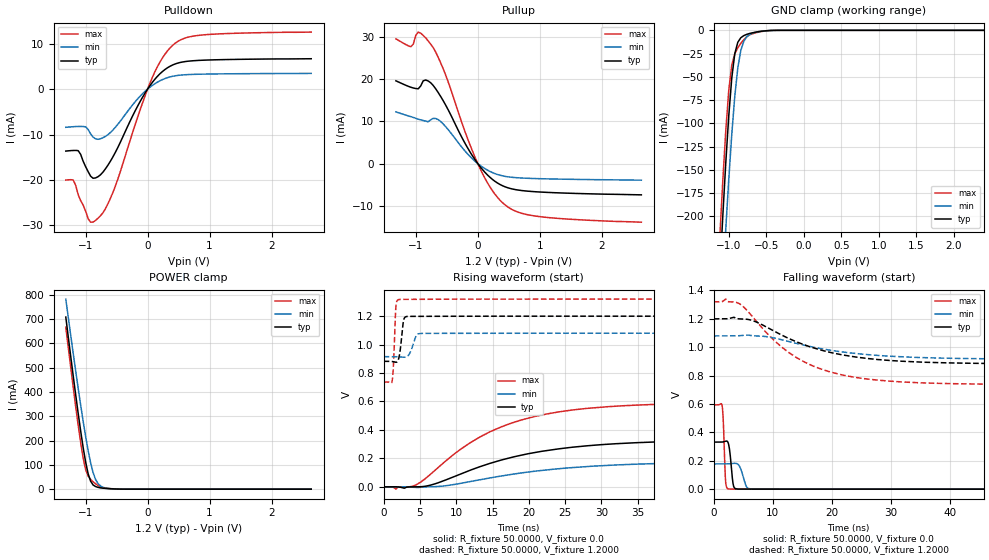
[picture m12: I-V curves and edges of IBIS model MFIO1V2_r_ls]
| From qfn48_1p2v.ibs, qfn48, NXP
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[Model] MFIO1V2_r_ls
|   Model MFIO1V2_r_ls
| This model was characterised for following simulation conditions:
| External (pad) voltage:
|   - Typ: 1.2V,   - Min: 1.08V,   - Max: 1.32V
| Library cells for typ/min/max conditions are connected as defined below:
|  IO - External Pad
|  A - Core Input
|  EN - Output Buffer Enable
|  BOOST - vdde
|  EHS - gnd
|  ENZI - vdd
|  EPD - vdd
|  EPUN - gnd
|  ZI - NC
|  ZIF - NC
|  gnd - gnd
|  gnde - gnde
|  vdd - vdd
|  vdde - vdde
| All other pins connected to ground
Model_type I/O
Polarity   Non-Inverting
Enable   Active-Low
Vinl =   0.3600V
Vinh =   0.8400V
Vmeas =  0.6000V
Cref =   20.0000F
Rref =   1.0000M
Vref =   0.0V
C_comp   1.6368pF   1.5495pF   1.7159pF
|C_comp_pullup   0.8309pF   0.8676pF   0.7830pF
|C_comp_pulldown   0.5929pF   0.6311pF   0.5574pF
[Model Spec]
| variable   typ   min   max
Vinh   0.3600V   0.3240V   0.3960V
Vinl   0.8400V   0.7560V   0.9240V
Vmeas   0.6000V   0.5400V   0.6600V
[Temperature Range]   25.0000   0.1250k   -40.0000
[Voltage Range]   1.2000V   1.0800V   1.3200V
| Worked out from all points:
|   slope of the pulldown table from 0 to 0.18 V, typ, clamps not added: 58.2 ohm
|   slope of the pullup table from 0 to 0.18 V, typ, clamps not added: 59.4 ohm
|   GND clamp passes 1 mA (typ) near -0.56 V on its own axis
|   POWER clamp passes 1 mA (typ) near -0.54 V on its own axis
|   rising waveform, R_fixture 50.0000, V_fixture 0.0: 20-80 % time 14.4ns typ, 16.1ns min, 12.2ns max; typ from 0 V to 0.331 V
|   rising waveform, R_fixture 50.0000, V_fixture 1.2000: 20-80 % time 407ps typ, 670ps min, 259ps max; typ from 0.882 V to 1.2 V
|   falling waveform, R_fixture 50.0000, V_fixture 0.0: 20-80 % time 465ps typ, 791ps min, 298ps max; typ from 0.331 V to 0 V
|   falling waveform, R_fixture 50.0000, V_fixture 1.2000: 20-80 % time 12.6ns typ, 13.9ns min, 10.9ns max; typ from 1.2 V to 0.882 V
[Pulldown]
|Voltage   I(typ)   I(min)   I(max)
-1.32V    -13.65mA   -8.413mA   -20.02mA
-1.2V     -13.51mA   -8.286mA   -20.01mA
-1.12V    -13.55mA   -8.228mA   -23.23mA
-920mV    -19.16mA   -9.849mA   -29.29mA
-720mV    -18.27mA   -10.7mA    -27.21mA
-520mV    -13.92mA   -8.406mA   -21.33mA
-160mV    -3.727mA   -2.148mA   -6.154mA
80mV      1.535mA    840.4uA    2.681mA
280mV     4.299mA    2.312mA    7.674mA
480mV     5.684mA    2.989mA    10.42mA
960mV     6.383mA    3.3mA      11.99mA
2.64V     6.67mA     3.446mA    12.53mA
[Pullup]
|Voltage   I(typ)   I(min)   I(max)
-1.32V    19.64mA    12.26mA    29.6mA
-1.08V    18.12mA    11.13mA    27.73mA
-960mV    17.74mA    10.54mA    31.21mA
-840mV    19.83mA    10.07mA    29.84mA
-720mV    18.57mA    10.71mA    27.56mA
-520mV    13.94mA    8.794mA    21.09mA
-200mV    4.663mA    2.883mA    7.362mA
40mV      -771.3uA   -452.7uA   -1.28mA
240mV     -3.804mA   -2.171mA   -6.507mA
480mV     -5.732mA   -3.143mA   -10.26mA
1.04V     -6.794mA   -3.614mA   -12.68mA
2.64V     -7.439mA   -3.951mA   -13.93mA
[GND_clamp]
|Voltage   I(typ)   I(min)   I(max)
-1.32V    -596.2mA   -647.7mA   -564.2mA
-1.12V    -261.7mA   -329.6mA   -222.8mA
-1.08V    -200.1mA   -270.2mA   -162.2mA
-1.04V    -142.4mA   -213.4mA   -108mA
-1V       -91.66mA   -160.1mA   -64.4mA
-960mV    -51.26mA   -111.8mA   -37.36mA
-920mV    -25.17mA   -71.04mA   -25.19mA
-880mV    -12.89mA   -40.68mA   -18.85mA
-800mV    -5.7mA     -11.79mA   -10.05mA
-680mV    -2.586mA   -2.926mA   -3.538mA
-440mV    -160.8uA   -186.1uA   -197.3uA
2.64V     0A         0A         0A
[POWER_clamp]
|Voltage   I(typ)   I(min)   I(max)
-1.32V    708.1mA    782.2mA    666.5mA
-1.2V     465.5mA    558mA      418.6mA
-1.12V    311.6mA    414.8mA    262.8mA
-1.04V    171.5mA    279.6mA    128.1mA
-1V       111.7mA    217mA      80.3mA
-960mV    64.07mA    159.3mA    53.87mA
-920mV    33.02mA    108.9mA    40.24mA
-880mV    17.44mA    68.44mA    30.42mA
-840mV    10.78mA    40.19mA    22.06mA
-760mV    5.295mA    13.21mA    9.362mA
-440mV    235.7uA    303.1uA    277.6uA
2.64V     0A         0A         0A
[Ramp]
| variable   typ   min   max
dV/dt_r  0.1988/14.4041n   0.1066/16.1004n   0.3561/12.2022n
dV/dt_f  0.1904/12.5637n   98.7976m/13.9154n   0.3496/10.8860n
R_load = 50.0000
[Rising Waveform]
R_fixture= 50.0000
V_fixture= 0.0
V_fixture_min= 0.0
V_fixture_max= 0.0
|time   V(typ)   V(min)   V(max)
0s        1.234nV    117.7nV    49.88pV
1.691ns   85.74uV    74.21uV    -16.49mV
4.659ns   -378.8uV   -5.08mV    18.94mV
6.853ns   17.36mV    563.8uV    106.2mV
10.6ns    90.24mV    24.23mV    264.1mV
16.16ns   187.6mV    75.83mV    420.6mV
20.77ns   240.4mV    109.5mV    493.7mV
26ns      278.3mV    135.2mV    539.8mV
43.95ns   323.2mV    169.9mV    586.8mV
100ns     331.4mV    177.6mV    593.5mV
[Rising Waveform]
R_fixture= 50.0000
V_fixture= 1.2000
V_fixture_min= 1.0800
V_fixture_max= 1.3200
|time   V(typ)   V(min)   V(max)
0s        882mV      914.8mV    736.7mV
1.168ns   880.6mV    915mV      743.8mV
1.364ns   878.7mV    915.1mV    868mV
1.68ns    875.4mV    914.4mV    1.262V
2.124ns   911.9mV    912.8mV    1.317V
2.752ns   1.171V     910.6mV    1.317V
3.279ns   1.198V     917.7mV    1.317V
4.498ns   1.198V     1.063V     1.317V
5.353ns   1.198V     1.078V     1.318V
100ns     1.199V     1.079V     1.319V
[Falling Waveform]
R_fixture= 50.0000
V_fixture= 0.0
V_fixture_min= 0.0
V_fixture_max= 0.0
|time   V(typ)   V(min)   V(max)
0s        331.4mV    177.7mV    593.5mV
1.416ns   331.7mV    177.7mV    586.5mV
1.616ns   333.4mV    177.6mV    474.7mV
1.984ns   337.6mV    177.5mV    62.87mV
2.558ns   306.3mV    178.4mV    1.331mV
3.31ns    27.54mV    181.5mV    677.8uV
4.043ns   997.4uV    176.9mV    790uV
5.564ns   562.7uV    15.2mV     575.5uV
6.583ns   522.7uV    931.9uV    432.4uV
100ns     11.27nV    159.8nV    8.885nV
[Falling Waveform]
R_fixture= 50.0000
V_fixture= 1.2000
V_fixture_min= 1.0800
V_fixture_max= 1.3200
|time   V(typ)   V(min)   V(max)
0s        1.199V     1.079V     1.319V
2.024ns   1.199V     1.079V     1.339V
4.347ns   1.199V     1.081V     1.306V
6.557ns   1.188V     1.081V     1.214V
10.26ns   1.112V     1.064V     1.045V
15.51ns   1.014V     1.012V     891.8mV
19.32ns   967mV      981.1mV    829.8mV
24.81ns   926.3mV    952.1mV    781.9mV
41.72ns   887.7mV    920.5mV    741.9mV
100ns     882mV      914.8mV    736.7mV
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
